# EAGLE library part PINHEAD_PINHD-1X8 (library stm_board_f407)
PIN HEADER
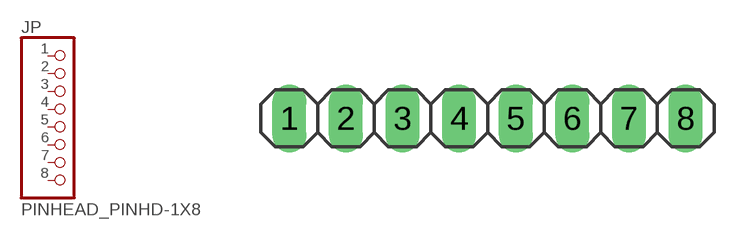
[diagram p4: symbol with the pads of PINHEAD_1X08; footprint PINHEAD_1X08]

Designator prefix JP

## PINHEAD_PINHD-1X8  [PINHEAD_1X08]
1  1  pas
2  2  pas
3  3  pas
4  4  pas
5  5  pas
6  6  pas
7  7  pas
8  8  pas

## Footprint PINHEAD_1X08 (pad centres in mm)
PIN HEADER
drill 1.016 long: 1 -8.89,0; 2 -6.35,0; 3 -3.81,0; 4 -1.27,0; 5 1.27,0; 6 3.81,0; 7 6.35,0; 8 8.89,0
